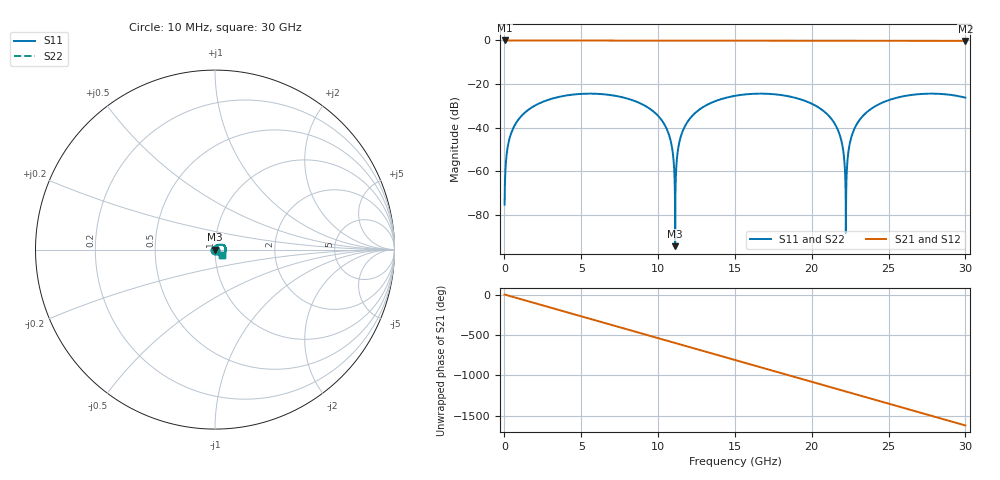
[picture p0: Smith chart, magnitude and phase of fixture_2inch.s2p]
! Created with skrf 1.10.0 (http://scikit-rf.org).
# Hz S RI R 50.0
!freq ReS11 ImS11 ReS21 ImS21 ReS12 ImS12 ReS22 ImS22
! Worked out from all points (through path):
!   3000 points, 10 MHz to 30 GHz, reference 50 ohm
!   highest |S21| = 0.00 dB at 10 MHz (marker M1); lowest = -0.2 dB at 30 GHz (marker M2)
!   group delay of S21, straight-line fit = 150 ps
!   lowest |S11| = -94.5 dB at 11.11 GHz (marker M3), VSWR 1.00, Z = 50 - j0.00188 ohm
!   |S11| at or under -10 dB: start of sweep to end of sweep
!   |S22| runs from -94.5 to -24.4 dB; largest |S21 - S12| = 0
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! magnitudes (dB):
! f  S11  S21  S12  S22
! 10 MHz  -75.4  0.0  0.0  -75.4
! 180 MHz  -50.3  0.0  0.0  -50.3
! 300 MHz  -45.9  0.0  0.0  -45.9
! 1.01 GHz  -35.4  0.0  0.0  -35.4
! 2.59 GHz  -27.9  0.0  0.0  -27.9
! 5.01 GHz  -24.5  -0.1  -0.1  -24.5
! 8.01 GHz  -26.7  -0.1  -0.1  -26.7
! 10.01 GHz  -34.7  -0.1  -0.1  -34.7
! 10.71 GHz  -43.4  -0.1  -0.1  -43.4
! 11.11 GHz  -94.5  -0.1  -0.1  -94.5
! 11.48 GHz  -44.1  -0.1  -0.1  -44.1
! 12.08 GHz  -35.8  -0.1  -0.1  -35.8
! 15.01 GHz  -25.4  -0.1  -0.1  -25.4
! 17.69 GHz  -24.8  -0.1  -0.1  -24.8
! 20.01 GHz  -29.1  -0.1  -0.1  -29.1
! 21.59 GHz  -39.4  -0.1  -0.1  -39.4
! 21.93 GHz  -46.1  -0.1  -0.1  -46.1
! 22.22 GHz  -88.5  -0.1  -0.1  -88.5
! 22.55 GHz  -45.1  -0.1  -0.1  -45.1
! 22.97 GHz  -38.0  -0.1  -0.1  -38.0
! 25.01 GHz  -27.4  -0.2  -0.2  -27.4
! 30 GHz  -26.3  -0.2  -0.2  -26.3
